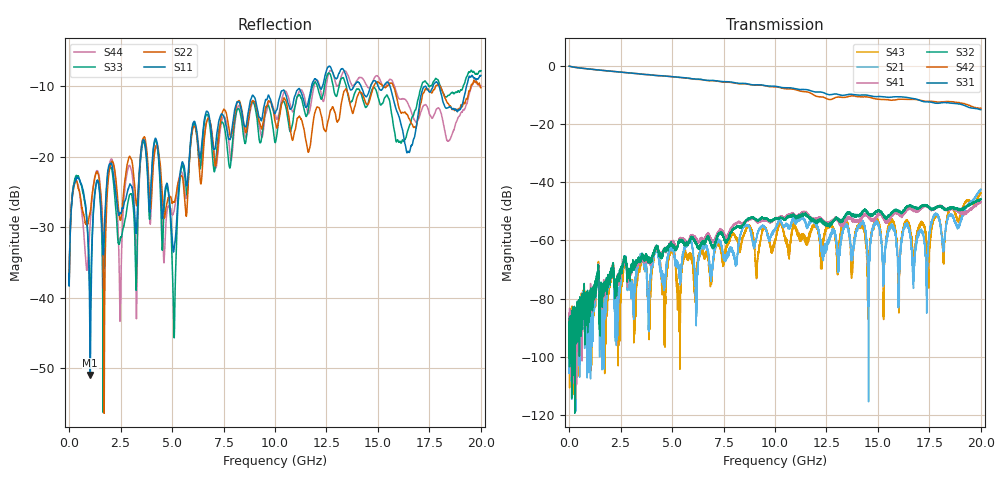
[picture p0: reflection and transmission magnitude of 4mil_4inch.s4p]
!Agilent Technologies,N5230A,US43500443,A.06.04.32
!Agilent N5230A: A.06.04.32
!Date: Wednesday, December 12, 2012 16:35:33
!Correction: S11(Full 4 Port(1,2,3,4)) S12(Full 4 Port(1,2,3,4)) S13(Full 4 Port(1,2,3,4)) S14(Full 4 Port(1,2,3,4)) S21(Full 4 Port(1,2,3,4)) S22(Full 4 Port(1,2,3,4)) S23(Full 4 Port(1,2,3,4)) S24(Full 4 Port(1,2,3,4)) S31(Full 4 Port(1,2,3,4)) S32(Full 4 Port(1,2,3,4)) S33(Full 4 Port(1,2,3,4)) S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
!S4P File: Measurements: <S11,S12,S13,S14>, <S21,S22,S23,S24>, <S31,S32,S33,S34>, <S41,S42,S43,S44>:
# Hz S  dB  R 50
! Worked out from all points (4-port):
!   10000 points, 1 MHz to 20 GHz, reference 50 ohm
!   strongest paths, dB at 1 MHz, 5.001 GHz, 10 GHz, 15 GHz, 20 GHz:
!     S31: -0.1, -3.7, -7.0, -10.6, -15.1
!     S42: -0.1, -3.7, -7.2, -11.5, -14.6
!     S32: -89.1, -61.4, -52.5, -49.7, -45.7
!     S41: -86.0, -60.1, -52.5, -51.0, -46.6
!     S21: -87.8, -62.2, -56.3, -54.7, -42.4
!     S43: -89.0, -64.3, -60.0, -53.1, -43.7
!   lowest |S11| = -51.0 dB at 1.027 GHz (marker M1), VSWR 1.01, Z = 49.8 + j0.238 ohm
!   |S11| at or under -10 dB: start of sweep to 11.77 GHz; 15.59 GHz to 17.28 GHz (1.689 GHz wide, 10.3 % of centre); 17.98 GHz to 19.3 GHz (1.323 GHz wide, 7.1 % of centre)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
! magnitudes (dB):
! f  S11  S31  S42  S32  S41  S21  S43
! 1 MHz  -36.6  -0.1  -0.1  -89.1  -86.0  -87.8  -89.0
! 1.027 GHz  -51.0  -1.1  -1.1  -79.6  -79.7  -92.7  -87.0
! 1.989 GHz  -21.0  -1.8  -1.8  -72.0  -73.1  -72.2  -73.9
! 5.097 GHz  -33.1  -3.7  -3.8  -61.8  -60.6  -64.0  -63.7
! 11.3 GHz  -11.1  -8.1  -8.7  -51.3  -50.3  -52.0  -59.4
! 16.73 GHz  -17.5  -11.2  -11.5  -48.5  -50.1  -72.6  -66.0
! 20 GHz  -8.4  -15.1  -14.6  -45.7  -46.6  -42.4  -43.7
